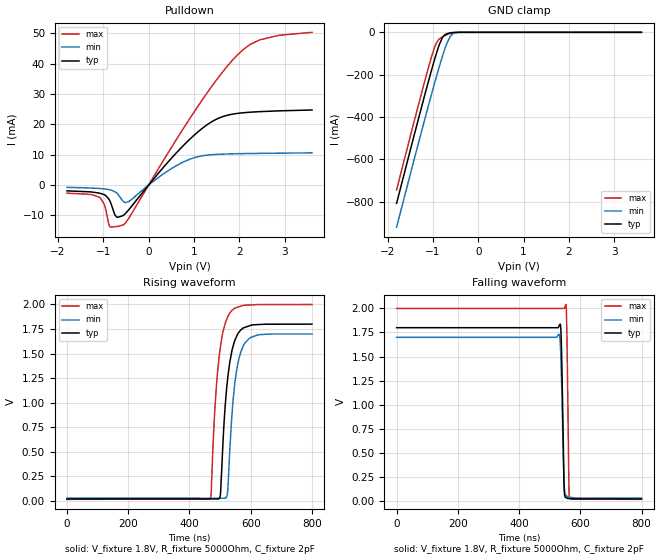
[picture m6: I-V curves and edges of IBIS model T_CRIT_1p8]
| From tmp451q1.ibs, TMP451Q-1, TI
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|   Model
[Model]   T_CRIT_1p8
Model_type   Open_drain
Polarity   Non-Inverting
Vmeas = 0.9
Vref = 1.8
Cref = 2pF
Rref = 5000
|   typ   min   max
C_comp   1.79pF   1.74pF   2pF
[Voltage Range]   1.8   1.7   2
[Temperature Range]   25   125   -40
[Pullup Reference]   1.8   1.7   2
[Pulldown Reference]   0   0   -0
[GND Clamp Reference]   0   0   0
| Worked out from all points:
|   slope of the pulldown table from 0 to 0.27 V, typ, clamps not added: 55.6 ohm
|   GND clamp passes 1 mA (typ) near -0.56 V on its own axis
|   falling waveform, V_fixture 1.8V, R_fixture 5000Ohm, C_fixture 2pF: 20-80 % time 6.08ns typ, 7.64ns min, 4.94ns max; typ from 1.8 V to 0.019 V
|   rising waveform, V_fixture 1.8V, R_fixture 5000Ohm, C_fixture 2pF: 20-80 % time 27.4ns typ, 27ns min, 27.7ns max; typ from 0.019 V to 1.8 V
[Pulldown]
|   Voltage   I(typ)   I(min)   I(max)
-1.8V     -1.928mA   -768.6uA   -2.68mA
-1.076V   -2.701mA   -1.157mA   -4.073mA
-973.8mV  -3.22mA    -1.298mA   -6.589mA
-855mV    -5.258mA   -1.572mA   -13.69mA
-703.8mV  -10.56mA   -2.64mA    -13.68mA
-541.8mV  -9.793mA   -5.625mA   -12.92mA
462.6mV   8.154mA    5.031mA    11.41mA
991.8mV   16.25mA    8.92mA     23.82mA
1.445V    21.3mA     10.04mA    33.59mA
1.948V    23.55mA    10.3mA     42.68mA
2.45V     24.16mA    10.42mA    47.8mA
3.6V      24.7mA     10.58mA    50.28mA
[GND Clamp]
|   Voltage   I(typ)   I(min)   I(max)
-1.8V     -808.6mA   -921mA     -744.9mA
-1.195V   -309.3mA   -424.2mA   -243.1mA
-1.039V   -185.9mA   -299.8mA   -121.8mA
-973.8mV  -136.9mA   -249.4mA   -77.6mA
-936mV    -109.6mA   -220.5mA   -56.19mA
-882mV    -73.11mA   -179.9mA   -36.1mA
-779.4mV  -21.83mA   -106.8mA   -20.69mA
-687.6mV  -6.414mA   -50.41mA   -10.56mA
-617.4mV  -2.588mA   -19.58mA   -4.826mA
-547.2mV  -715.7uA   -4.874mA   -1.318mA
-363.6mV  -2.267uA   -42.71uA   -1.028uA
3.6V      0A         0A         0A
[Ramp]
R_load = 5000
|   typ   min   max
dV/dt_r   1.06838/2.71832e-08   1.00325/2.67966e-08   1.19052/2.76905e-08
dV/dt_f   1.06838/6.07586e-09   1.00325/7.6427e-09   1.19052/4.93512e-09
[Falling Waveform]
V_fixture = 1.8V
V_fixture_min = 1.7V
V_fixture_max = 2V
R_fixture = 5000Ohm
C_fixture = 2pF
|   Time   V(typ)   V(min)   V(max)
0s        1.8V       1.7V       2V
531ns     1.82V      1.732V     2V
534.8ns   1.836V     1.625V     2V
538.7ns   1.57V      1.249V     2V
547.4ns   131.1mV    167.2mV    2V
553.2ns   33.04mV    55.64mV    2.041V
556.2ns   28.8mV     46.56mV    1.724V
562.9ns   24.08mV    38.08mV    146mV
565ns     23.6mV     37.32mV    30.54mV
800ns     19.37mV    27.91mV    15.8mV
[Rising Waveform]
V_fixture = 1.8V
V_fixture_min = 1.7V
V_fixture_max = 2V
R_fixture = 5000Ohm
C_fixture = 2pF
|   Time   V(typ)   V(min)   V(max)
0s        19.37mV    27.91mV    15.8mV
467ns     20.43mV    27.37mV    18.62mV
471ns     20.44mV    27.36mV    88.19mV
486.6ns   20.48mV    27.35mV    1.109V
500.3ns   46.99mV    27.33mV    1.551V
513.9ns   843.8mV    27.31mV    1.775V
525.6ns   1.271V     133.1mV    1.88V
547.7ns   1.631V     1.188V     1.962V
576.5ns   1.762V     1.584V     1.992V
800ns     1.8V       1.7V       2V
